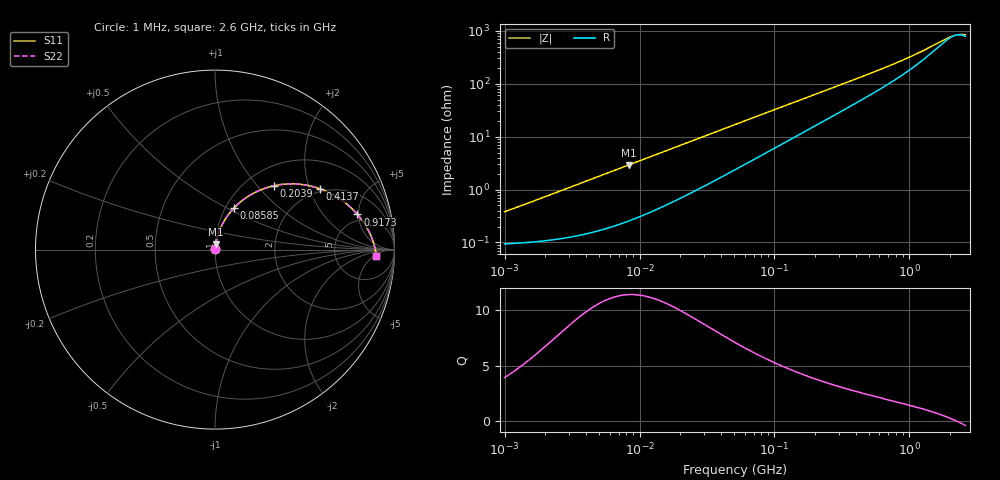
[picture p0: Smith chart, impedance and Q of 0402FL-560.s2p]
# MHz S MA R 50
!Freq  MagS11  AngS11  MagS21  AngS21  MagS12  AngS12  MagS22  AngS22
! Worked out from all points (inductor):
!   801 points, 1 MHz to 2.6 GHz, reference 50 ohm
!   read as one part in series: L = 58.3 nH near 1.04 MHz
!   highest Q = 11.4 at 8.357 MHz (marker M1), where L = 55.5 nH
!   self-resonance near 2.248 GHz
!   S11 on the Smith chart (normalised r, x): 1 MHz: 1.00, +0.01; 85.85 MHz: 1.10, +0.55; 203.9 MHz: 1.33, +1.24; 413.7 MHz: 1.90, +2.37; 917.3 MHz: 4.10, +4.84; 2.6 GHz: 17, -6
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1  0.003801 75.5  0.9991 -0.2  0.9991 -0.2  0.003801 75.5
1.410604  0.005246 78.8  0.999 -0.3  0.999 -0.3  0.005246 78.8
3.732571  0.01336 83.3  0.9985 -0.8  0.9985 -0.8  0.01336 83.3
8.356854  0.02917 83.3  0.997 -1.7  0.997 -1.7  0.02917 83.3
13.79581  0.04735 82.1  0.9946 -2.7  0.9946 -2.7  0.04735 82.1
27.72211  0.09232 78.4  0.9856 -5.3  0.9856 -5.3  0.09232 78.4
50.9902  0.1628 72.7  0.9642 -9.3  0.9642 -9.3  0.1628 72.7
67.14455  0.2083 69.1  0.9459 -11.9  0.9459 -11.9  0.2083 69.1
85.8477  0.2574 65.3  0.9225 -14.7  0.9225 -14.7  0.2574 65.3
127.1971  0.3524 57.9  0.8657 -20.2  0.8657 -20.2  0.3524 57.9
190.3245  0.4654 48.8  0.7771 -26.8  0.7771 -26.8  0.4654 48.8
203.8805  0.4854 47.2  0.7589 -28.0  0.7589 -28.0  0.4854 47.2
290.4354  0.5864 38.5  0.6528 -34.0  0.6528 -34.0  0.5864 38.5
413.736  0.6766 30.0  0.5348 -39.3  0.5348 -39.3  0.6766 30.0
539.4841  0.7333 24.1  0.446 -42.2  0.446 -42.2  0.7333 24.1
703.4513  0.7799 18.7  0.3618 -43.8  0.3618 -43.8  0.7799 18.7
917.2535  0.8174 13.9  0.2846 -43.5  0.2846 -43.5  0.8174 13.9
1345.765  0.8582 7.6  0.1881 -37.4  0.1881 -37.4  0.8582 7.6
1807.302  0.8807 3.2  0.1305 -22.3  0.1305 -22.3  0.8807 3.2
2013.663  0.8873 1.6  0.1159 -12.6  0.1159 -12.6  0.8873 1.6
2288.127  0.8938 -0.3  0.1063 2.3  0.1063 2.3  0.8938 -0.3
2600  0.8991 -2.2  0.1073 18.8  0.1073 18.8  0.8991 -2.2
